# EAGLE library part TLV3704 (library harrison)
COMPARATOR
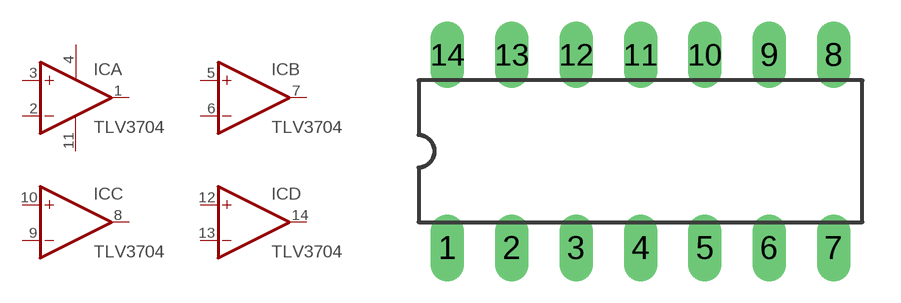
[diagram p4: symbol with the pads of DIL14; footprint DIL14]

Designator prefix IC; gates A=OPAMP B=OPAMP C=OPAMP D=OPAMP P=PWR+-

## TLV3704  [DIL14]
1  A:OUT  out
2  A:-IN  in
3  A:+IN  in
4  P:V+  pwr
5  B:+IN  in
6  B:-IN  in
7  B:OUT  out
8  C:OUT  out
9  C:-IN  in
10  C:+IN  in
11  P:V-  pwr
12  D:+IN  in
13  D:-IN  in
14  D:OUT  out

## Footprint DIL14 (pad centres in mm)
drill 0.813 long: 1 -7.62,-3.81; 2 -5.08,-3.81; 3 -2.54,-3.81; 4 0,-3.81; 5 2.54,-3.81; 6 5.08,-3.81; 7 7.62,-3.81; 8 7.62,3.81; 9 5.08,3.81; 10 2.54,3.81; 11 0,3.81; 12 -2.54,3.81; 13 -5.08,3.81; 14 -7.62,3.81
